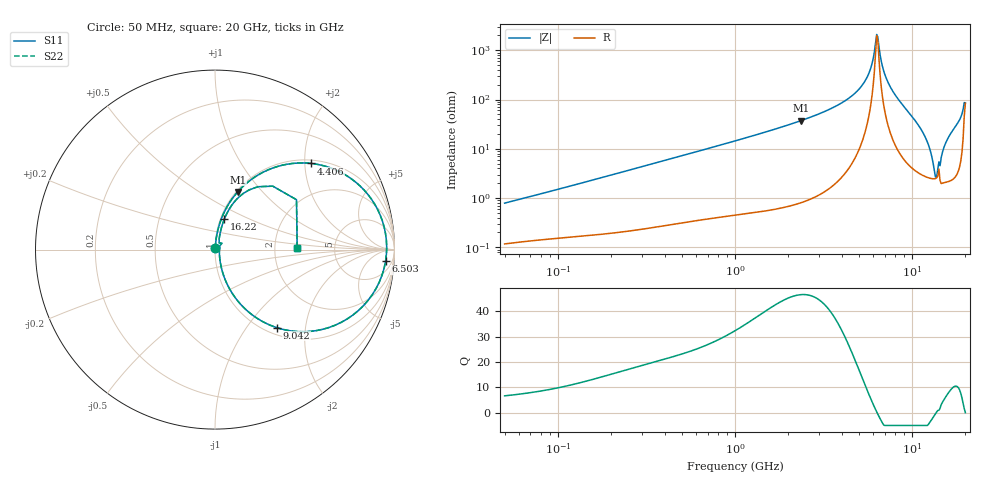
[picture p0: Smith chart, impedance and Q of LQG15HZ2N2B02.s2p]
!Murata Part Number: LQG15HZ2N2B02
!These Parameters are Measured in Series Mode Connection
!  o--[Z]--o
!Port1  Port2
!  o-------o
!Freq. Start=50[MHz] Stop=20[GHz], 401[Steps]
# Hz S RI R 50
!Freq.(Hz) S11(Real) S11(Imag) S21(Real) S21(Imag) S12(Real) S12(Imag) S22(Real) S22(Imag)
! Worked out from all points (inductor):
!   401 points, 50 MHz to 20 GHz, reference 50 ohm
!   read as one part in series: L = 2.44 nH near 51.52 MHz
!   highest Q = 46.5 at 2.349 GHz (marker M1), where L = 2.52 nH
!   self-resonance near 6.312 GHz
!   S11 on the Smith chart (normalised r, x): 50 MHz: 1.00, +0.02; 4.406 GHz: 1.08, +2.14; 6.503 GHz: 14, -20; 9.042 GHz: 1.12, -1.40; 16.22 GHz: 1.04, +0.36; 20 GHz: 2.69, +0.08
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5e7  0.00123 0.00777  0.9988 -0.00777  0.9988 -0.00777  0.00123 0.00777
1.364002e8  0.00208 0.0201  0.9979 -0.0201  0.9979 -0.0201  0.00208 0.0201
3.721004e8  0.00549 0.0534  0.9945 -0.0534  0.9945 -0.0534  0.00549 0.0534
1e9  0.0246 0.1402  0.9754 -0.1402  0.9754 -0.1402  0.0246 0.1402
2.348516e9  0.1265 0.3218  0.8735 -0.3218  0.8735 -0.3218  0.1265 0.3218
2.728004e9  0.1748 0.3691  0.8252 -0.3691  0.8252 -0.3691  0.1748 0.3691
4.405649e9  0.5337 0.4802  0.4663 -0.4802  0.4663 -0.4802  0.5337 0.4802
5.433528e9  0.8315 0.331  0.1685 -0.331  0.1685 -0.331  0.8315 0.331
5.856089e9  0.9197 0.194  0.0803 -0.194  0.0803 -0.194  0.9197 0.194
6.217679e9  0.9548 0.0523  0.0452 -0.0523  0.0452 -0.0523  0.9548 0.0523
6.503449e9  0.9504 -0.0643  0.0496 0.0643  0.0496 0.0643  0.9504 -0.0643
6.905011e9  0.8981 -0.2156  0.1019 0.2156  0.1019 0.2156  0.8981 -0.2156
7.442007e9  0.7677 -0.365  0.2323 0.365  0.2323 0.365  0.7677 -0.365
9.041845e9  0.3437 -0.4347  0.6563 0.4347  0.6563 0.4347  0.3437 -0.4347
1.166392e10  0.0607 -0.177  0.9393 0.177  0.9393 0.177  0.0607 -0.177
1.257102e10  0.0335 -0.0921  0.9665 0.0921  0.9665 0.0921  0.0335 -0.0921
1.354865e10  0.0243 -0.00961  0.9757 0.00961  0.9757 0.00961  0.0243 -0.00961
1.396067e10  0.0278 0.0233  0.9722 -0.0233  0.9722 -0.0233  0.0278 0.0233
1.527346e10  0.0325 0.1091  0.9675 -0.1091  0.9675 -0.1091  0.0325 0.1091
1.621653e10  0.0514 0.1687  0.9486 -0.1687  0.9486 -0.1687  0.0514 0.1687
1.88369e10  0.1901 0.3326  0.8099 -0.3326  0.8099 -0.3326  0.1901 0.3326
2e10  0.4579 0.0112  0.5421 -0.0112  0.5421 -0.0112  0.4579 0.0112
